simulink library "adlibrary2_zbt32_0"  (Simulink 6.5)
undefined symbols (not defined in the file or in its folder): Black, blackbox2, blue, Box, gcbh, Inactive, VER_STRING_GOES_HERE, white, xbsIndex_r4, xlBlockLoadCallback, zbt32_config
libraries: xbsIndex_r4 x16, adlibrary2_zbt32_0 x1

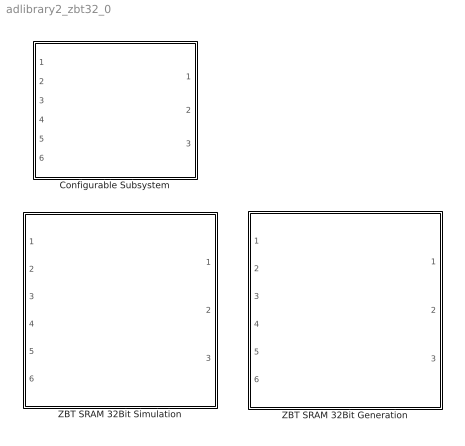
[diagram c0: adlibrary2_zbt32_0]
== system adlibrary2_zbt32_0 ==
  Configurable Subsystem : Subsystem  Tag=configX  BlockChoice=ZBT SRAM 32Bit Generation
  ZBT SRAM 32Bit Generation : Subsystem
  ZBT SRAM 32Bit Simulation : Subsystem

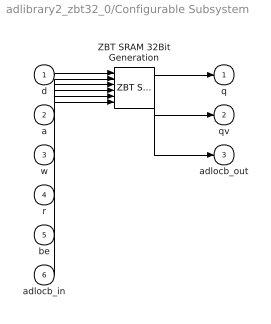
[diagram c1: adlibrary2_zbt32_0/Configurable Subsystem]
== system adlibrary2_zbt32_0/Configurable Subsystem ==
  d : Inport
  a : Inport  Port=2
  w : Inport  Port=3
  r : Inport  Port=4
  be : Inport  Port=5
  adlocb_in : Inport  Port=6
  ZBT SRAM 32Bit Generation : adlibrary2_zbt32_0/ZBT SRAM 32Bit Generation  SystemSampleTime=-1
  q : Outport
  qv : Outport  Port=2
  adlocb_out : Outport  Port=3
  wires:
  d/1 -> ZBT SRAM 32Bit Generation/1
  a/1 -> ZBT SRAM 32Bit Generation/2
  w/1 -> ZBT SRAM 32Bit Generation/3
  r/1 -> ZBT SRAM 32Bit Generation/4
  be/1 -> ZBT SRAM 32Bit Generation/5
  adlocb_in/1 -> ZBT SRAM 32Bit Generation/6
  ZBT SRAM 32Bit Generation/1 -> q/1
  ZBT SRAM 32Bit Generation/2 -> qv/1
  ZBT SRAM 32Bit Generation/3 -> adlocb_out/1

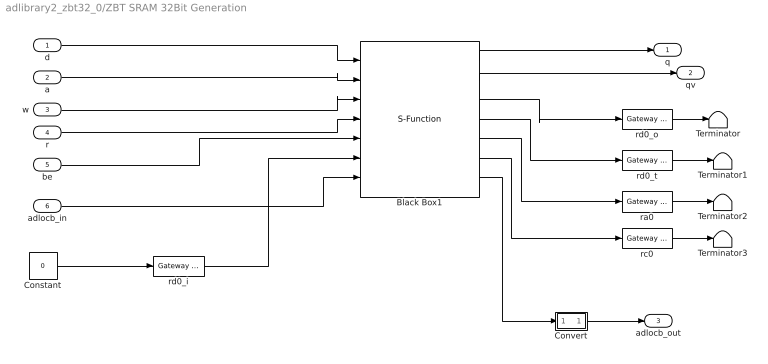
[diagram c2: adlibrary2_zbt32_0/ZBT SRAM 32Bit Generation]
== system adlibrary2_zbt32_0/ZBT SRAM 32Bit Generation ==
  d : Inport
  a : Inport  Port=2
  w : Inport  Port=3
  r : Inport  Port=4
  be : Inport  Port=5
  adlocb_in : Inport  Port=6
  Black Box1 : S-Function  AncestorBlock=xbsIndex_r4/Black Box  LoadFcn=xlBlockLoadCallback(gcbh);  FunctionName=sysgen  Parameters=ptable_  mask(Xilinx Black Box Block){infoedit=Incorporates black box HDL and simulation model into a System Generator design.<P><P>You must supply a Black Box with certain information about the HDL component you would like to bring into System Generator. This information is provided through a Matlab function.<P><P>When "Simulation mode" is set to "Inactive", you will typically want to provide a separate simulation model by using a Simulation 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, init_code=zbt32_config, sim_method=Inactive, sim_method_sgadvanced=, engine_block=, xl_use_area=off, xl_use_area_sgadvanced=, xl_area=[0,0,0,0,0,0,0], block_version=VER_STRING_GOES_HERE, has_advanced_control=0, sggui_pos=20,20,356,367, block_type=blackbox2, sg_icon_stat=130,170,7,7,white,blue,0,1b6b346b, sg_mask_display=fprintf('','COMMENT: begin icon graphics '); patch([0 130 130 0 ],[0 0 170 170 ],[0.77 0.82 0.91]); patch([31 9 39 9 31 65 74 83 120 91 63 43 74 43 63 91 120 83 74 65 31 ],[34 56 86 116 138 138 129 138 138 109 137 117 86 55 35 63 34 34 43 34 34 ],[0.98 0.96 0.92]); plot([0 0 130 130 0 ],[0 170 170 0 0 ]); fprintf('','COMMENT: end icon graphics');  fprintf('','COMMENT: begin icon text '); color('bl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, sg_list_contents=, adlocb_devid=0}
      mask prompts: infoedit ""; init_code "Block configuration m-function"; sim_method "Simulation mode"; engine_block "HDL co-simulator to use  (specify helper block by name)"; xl_use_area "Define FPGA area for resource estimation"; xl_area "FPGA area [slices, FFs, BRAMs, LUTs, IOBs, emb. mults, TBUFs]"; block_version ""; has_advanced_control ""; sggui_pos ""; block_type ""; sg_icon_stat ""; sg_mask_display ""; sg_list_contents ""; adlocb_devid "ADLOCB DEV ID"
      mask help: Incorporates black box HDL and simulation model into a System Generator design. You must supply a Black Box with certain information about the HDL component you would like to bring into System Generator. This information is provided through a Matlab function. When "Simulation mode" is set to "Inactive", you will typically want to provide a separate simulation model by using a Simulation Multiplexer. When "Simulation mode" is set to "External co-simulator", you must include a ModelSim block in the design.
      mask init:
      | xlMungeMaskParams;
      | 
      | mdlPath = xlGetMdlDir(bdroot);
      | 
      | refBlk = get_param(gcb,'referenceBlock');
      | if (isempty(refBlk) | strncmp(refBlk,'xbsIndex',8))
      | srcPath = mdlPath;
      | else
      | srcPath = xlPathToReference;
      | if (isempty(srcPath))
      | srcPath = mdlPath;
      | end
      | end
      | 
      | if (sim_method==3)
      | validEngineBlock = 0;
      | try
      | engineBlock = xlBlockNameRelPath(get_param(gcb,'Parent'),engine_block);
      | catch
      | engineBlock = '//';
      | end
      | try 
      | engineWorkDir = get_param(engineBlock,'dir');
      | validEngineBlock = 1;
      | engine_handle = get_param(engineBlock,'Handle');
      | catch
      | end
      | end
      | 
      | % build black box config function
      | block_config = ['sysgen:black_box_config:' init_code];
      | 
      | serialized_declarations = '{''engine_handle''=>''Double'',''sim_method''=>''Int'',''validEngineBlock''=>''Int'',''engineWorkDir''=>''String'',''engine_block''=>''String'',''init_code''=>''String'',''mdlPath''=>''String'',''srcPath''=>''String'',''block_config''=>''String'',}';
      | ptable_ = xlblockprep(get_param(gcb, 'MaskWSVariables'));
  Constant : Constant  Value=0  OutDataType=sfix(16)  ConRadixGroup=Use specified scaling  OutScaling=2^0  SampleTime=inf  FramePeriod=inf
  Convert : Subsystem
  Terminator{,1..3} (4 alike) : Terminator
  ra0 : xbsIndex_r4/Gateway Out  hdl_port=on  timing_constraint=None  locs_specified=off  LOCs={}  block_type=gatewayout
  rc0 : xbsIndex_r4/Gateway Out  hdl_port=on  timing_constraint=None  locs_specified=off  LOCs={}  block_type=gatewayout
  rd0_i : xbsIndex_r4/Gateway In  arith_type=Unsigned  n_bits=32  bin_pt=0  quantization="Round  (unbiased: +/- Inf)"  overflow=Saturate  period=ad_get_simulink_period  dbl_ovrd=off  timing_constraint=None  locs_specified=off  LOCs={}  block_type=gatewayin
  rd0_o : xbsIndex_r4/Gateway Out  hdl_port=on  timing_constraint=None  locs_specified=off  LOCs={}  block_type=gatewayout
  rd0_t : xbsIndex_r4/Gateway Out  hdl_port=on  timing_constraint=None  locs_specified=off  LOCs={}  block_type=gatewayout
  q : Outport
  qv : Outport  Port=2
  adlocb_out : Outport  Port=3
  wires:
  Convert/1(out0) -> adlocb_out/1
  Black Box1/7 -> Convert/1(in0)
  adlocb_in/1 -> Black Box1/7
  be/1 -> Black Box1/5
  rd0_i/1 -> Black Box1/6
  d/1 -> Black Box1/1
  Black Box1/1 -> q/1
  Black Box1/2 -> qv/1
  Constant/1 -> rd0_i/1
  rd0_o/1 -> Terminator/1
  rd0_t/1 -> Terminator1/1
  ra0/1 -> Terminator2/1
  rc0/1 -> Terminator3/1
  a/1 -> Black Box1/2
  w/1 -> Black Box1/3
  r/1 -> Black Box1/4
  Black Box1/3 -> rd0_o/1
  Black Box1/4 -> rd0_t/1
  Black Box1/5 -> ra0/1
  Black Box1/6 -> rc0/1

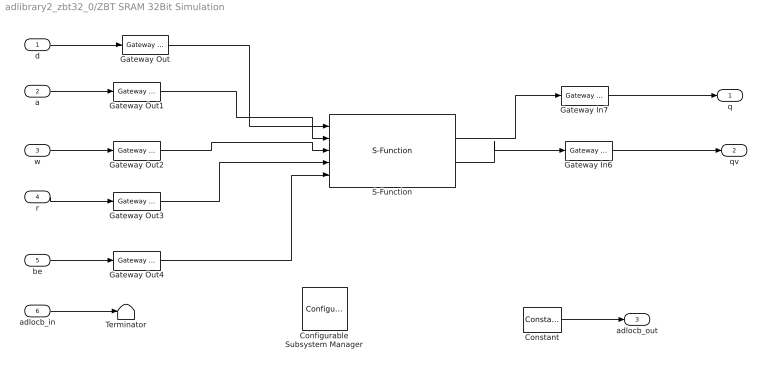
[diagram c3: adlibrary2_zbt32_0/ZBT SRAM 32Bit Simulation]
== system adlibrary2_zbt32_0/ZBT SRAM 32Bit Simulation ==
  d : Inport
  a : Inport  Port=2
  w : Inport  Port=3
  r : Inport  Port=4
  be : Inport  Port=5
  adlocb_in : Inport  Port=6
  Configurable Subsystem Manager : xbsIndex_r4/Configurable Subsystem Manager  Tag=xcfgMgr  block_type=configsubsys
  Constant : xbsIndex_r4/Constant  arith_type=Unsigned  const=0  n_bits=34  bin_pt=0  explicit_period=on  period=ad_get_simulink_period  equ=P=C  opselect=C  inp2=PCIN>>17  opr=+  inp1=P  carry=CIN  dbl_ovrd=off  block_type=constant
  Gateway In6 : xbsIndex_r4/Gateway In  arith_type=Boolean  n_bits=1  bin_pt=0  quantization="Round  (unbiased: +/- Inf)"  overflow=Saturate  period=ad_get_simulink_period  dbl_ovrd=on  timing_constraint=None  locs_specified=off  LOCs={}  block_type=gatewayin
  Gateway In7 : xbsIndex_r4/Gateway In  arith_type=Unsigned  n_bits=32  bin_pt=0  quantization="Round  (unbiased: +/- Inf)"  overflow=Saturate  period=ad_get_simulink_period  dbl_ovrd=on  timing_constraint=None  locs_specified=off  LOCs={}  block_type=gatewayin
  Gateway Out{,1..4} (5 alike) : xbsIndex_r4/Gateway Out  hdl_port=off  timing_constraint=None  locs_specified=off  LOCs={}  block_type=gatewayout
  S-Function : S-Function  FunctionName=zbt32  Parameters=0
  Terminator : Terminator
  q : Outport
  qv : Outport  Port=2
  adlocb_out : Outport  Port=3
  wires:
  be/1 -> Gateway Out4/1
  Gateway Out4/1 -> S-Function/5
  d/1 -> Gateway Out/1
  a/1 -> Gateway Out1/1
  w/1 -> Gateway Out2/1
  r/1 -> Gateway Out3/1
  S-Function/1 -> Gateway In7/1
  Gateway Out/1 -> S-Function/1
  Gateway Out1/1 -> S-Function/2
  Gateway Out2/1 -> S-Function/3
  Gateway Out3/1 -> S-Function/4
  Gateway In6/1 -> qv/1
  Gateway In7/1 -> q/1
  S-Function/2 -> Gateway In6/1
  Constant/1 -> adlocb_out/1
  adlocb_in/1 -> Terminator/1

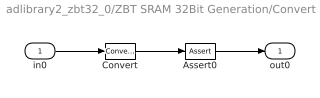
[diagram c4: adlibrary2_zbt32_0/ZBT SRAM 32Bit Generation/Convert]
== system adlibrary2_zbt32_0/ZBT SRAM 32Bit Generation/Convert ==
  in0 : Inport
  Assert0 : xbsIndex_r4/Assert  assert_type=off  type_source=Explicitly  arith_type="Signed  (2's comp)"  n_bits=16  bin_pt=14  assert_rate=on  rate_source=Explicitly  period=ad_get_simulink_period  output_port=on  block_type=assert
  Convert : xbsIndex_r4/Convert  arith_type=Unsigned  n_bits=34  bin_pt=0  quantization=Truncate  overflow=Wrap  latency=0  dbl_ovrd=off  pipeline=off  block_type=convert
  out0 : Outport
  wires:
  Assert0/1 -> out0/1
  Convert/1 -> Assert0/1
  in0/1 -> Convert/1
